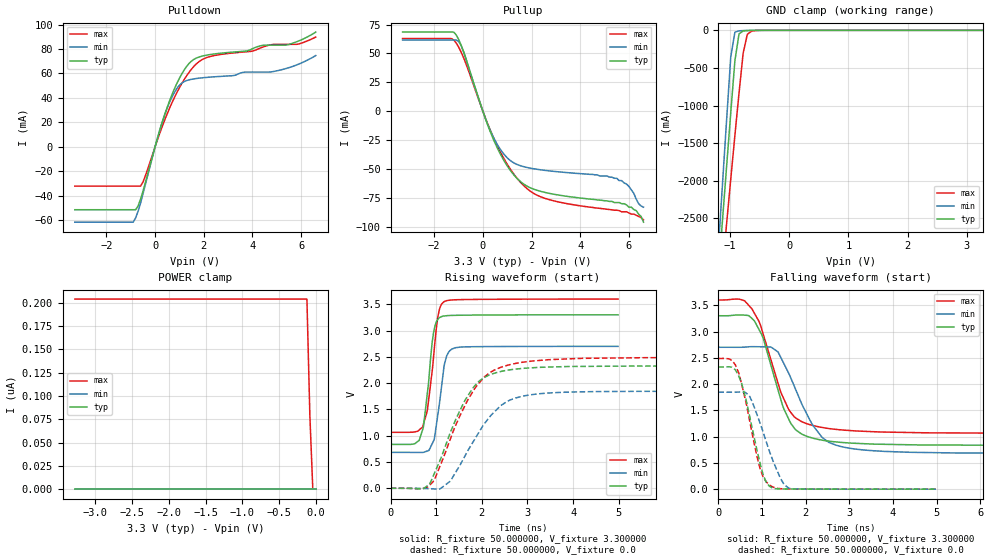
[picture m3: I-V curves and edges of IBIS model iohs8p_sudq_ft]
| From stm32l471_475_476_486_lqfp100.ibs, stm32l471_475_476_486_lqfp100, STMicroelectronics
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|   Model iohs8p_sudq_ft
[Model]  iohs8p_sudq_ft
Model_type I/O
Polarity   Non-Inverting
Enable   Active-Low
Vinl =   0.990000V
Vinh =   2.310000V
Vmeas =  1.650000V
Cref =   30.000000pF
Rref =   100.000000M
Vref =   0.0V
C_comp   2.036400pF   1.984000pF   2.082300pF
[Temperature Range]   25.000000   -40.000000   0.125000k
[Pullup Reference]   3.300000V   2.700000V   3.600000V
[Pulldown Reference]   0.0V   0.0V   0.0V
[POWER Clamp Reference]   3.300000V   2.700000V   3.600000V
[GND Clamp Reference]   0.0V   0.0V   0.0V
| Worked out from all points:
|   slope of the pulldown table from 0 to 0.495 V, typ, clamps not added: 15.4 ohm
|   slope of the pullup table from 0 to 0.495 V, typ, clamps not added: 18.1 ohm
|   GND clamp passes 1 mA (typ) near -0.60 V on its own axis
|   rising waveform, R_fixture 50.000000, V_fixture 3.300000: 20-80 % time 175ps typ, 184ps min, 191ps max; typ from 0.835 V to 3.3 V
|   rising waveform, R_fixture 50.000000, V_fixture 0.0: 20-80 % time 718ps typ, 830ps min, 808ps max; typ from 0 V to 2.33 V
|   falling waveform, R_fixture 50.000000, V_fixture 3.300000: 20-80 % time 564ps typ, 726ps min, 605ps max; typ from 3.3 V to 0.835 V
|   falling waveform, R_fixture 50.000000, V_fixture 0.0: 20-80 % time 381ps typ, 476ps min, 388ps max; typ from 2.33 V to 0 V
[Pulldown]
|Voltage   I(typ)   I(min)   I(max)
-3.3V     -51.63mA   -61.84mA   -32.32mA
-900mV    -51.63mA   -61.84mA   -32.32mA
-800mV    -51.63mA   -58.24mA   -32.32mA
-500mV    -36.51mA   -38.71mA   -28.96mA
400mV     26.66mA    26.58mA    22.18mA
800mV     47.72mA    44.74mA    40.6mA
1.1V      59.79mA    52.18mA    51.93mA
1.5V      70.22mA    55.24mA    63.66mA
2.1V      74.97mA    56.75mA    72.88mA
4.9V      83.19mA    61.75mA    83.83mA
5.9V      86.64mA    67.67mA    84.15mA
6.6V      93.9mA     74.68mA    89.84mA
[Pullup]
|Voltage   I(typ)   I(min)   I(max)
-3.3V     68.52mA    61.65mA    62.96mA
-1.1V     66.11mA    61.65mA    59.23mA
-800mV    51.99mA    51.74mA    46.62mA
100mV     -6.166mA   -5.972mA   -5.649mA
600mV     -32.08mA   -29.08mA   -30.29mA
1.2V      -53.2mA    -43.76mA   -52.32mA
1.9V      -65.77mA   -49.03mA   -68.4mA
3.1V      -72.48mA   -52.41mA   -78.44mA
5.5V      -79mA      -58mA      -85.6mA
6V        -83mA      -65mA      -88mA
6.3V      -86mA      -76mA      -90mA
6.6V      -96mA      -83mA      -94mA
[GND_clamp]
|Voltage   I(typ)   I(min)   I(max)
-3.3V     -9.812A    -9.822A    -9.937A
-1.2V     -3.251A    -2.905A    -3.763A
-1.13V    -2.527A    -2.046A    -3.165A
-1.06V    -1.808A    -1.191A    -2.57A
-990mV    -1.097A    -352.6mA   -1.979A
-920mV    -404.2mA   -25.08mA   -1.398A
-850mV    -46.53mA   -6.503mA   -832.3mA
-780mV    -8.496mA   -3.578mA   -302.4mA
-710mV    -3.383mA   -1.716mA   -53.8mA
-640mV    -1.589mA   -553.8uA   -11.72mA
-360mV    -2.023uA   0A         -84.67uA
3.28V     0A         0A         0A
[POWER_clamp]
|Voltage   I(typ)   I(min)   I(max)
-3.28V    0A         0A         204.1nA
-120mV    0A         0A         204.1nA
-80mV     0A         0A         79.47nA
-40mV     0A         0A         0A
0V        0A         0A         0A
[Ramp]
| variable   typ   min   max
dV/dt_r  1.39476/0.71674n   1.10718/0.82878n   1.49076/0.80690n
dV/dt_f  1.47901/0.56356n   1.21004/0.72569n   1.52124/0.60476n
R_load = 50.000000
[Rising Waveform]
R_fixture= 50.000000
V_fixture= 3.300000
V_fixture_min= 2.700000
V_fixture_max= 3.600000
|time   V(typ)   V(min)   V(max)
0s        835mV      683.3mV    1.065V
530.5ps   848.1mV    682.1mV    1.073V
700.7ps   1.11V      682.9mV    1.164V
810.8ps   1.844V     710.6mV    1.513V
940.9ps   2.954V     899mV      2.484V
1.041ns   3.221V     1.431V     3.281V
1.171ns   3.277V     2.318V     3.549V
1.281ns   3.286V     2.6V       3.577V
1.532ns   3.292V     2.686V     3.589V
4.985ns   3.3V       2.7V       3.6V
[Rising Waveform]
R_fixture= 50.000000
V_fixture= 0.0
V_fixture_min= 0.0
V_fixture_max= 0.0
|time   V(typ)   V(min)   V(max)
0s        24.38uV    -1.232uV   39.9uV
734.1ps   1.035mV    -3.343mV   -313.8uV
934.3ps   232.5mV    -11.62mV   128.5mV
1.101ns   566.2mV    -1.634mV   458.9mV
1.301ns   1.044V     130.8mV    917.4mV
1.602ns   1.625V     568.3mV    1.524V
1.902ns   2.007V     1.016V     1.962V
2.402ns   2.22V      1.563V     2.296V
2.803ns   2.273V     1.731V     2.385V
16.62ns   2.325V     1.845V     2.485V
[Falling Waveform]
R_fixture= 50.000000
V_fixture= 3.300000
V_fixture_min= 2.700000
V_fixture_max= 3.600000
|time   V(typ)   V(min)   V(max)
0s        3.3V       2.7V       3.6V
600.6ps   3.311V     2.703V     3.586V
834.2ps   3.192V     2.711V     3.336V
1.034ns   2.857V     2.709V     2.933V
1.368ns   1.888V     2.611V     2.016V
1.768ns   1.132V     1.904V     1.356V
2.336ns   938.9mV    1.031V     1.181V
2.936ns   882.5mV    789.5mV    1.12V
4.371ns   845.1mV    702.1mV    1.078V
16.62ns   835mV      683.3mV    1.065V
[Falling Waveform]
R_fixture= 50.000000
V_fixture= 0.0
V_fixture_min= 0.0
V_fixture_max= 0.0
|time   V(typ)   V(min)   V(max)
0s        2.325V     1.845V     2.485V
310.3ps   2.32V      1.845V     2.45V
450.5ps   2.187V     1.847V     2.245V
710.7ps   1.414V     1.775V     1.331V
951ps     511.3mV    1.267V     407.6mV
1.031ns   264.5mV    1.075V     230.5mV
1.181ns   51.28mV    698.8mV    72.53mV
1.431ns   5.2mV      195.2mV    8.721mV
1.622ns   3.374mV    16.99mV    4.414mV
4.985ns   24.38uV    -1.232uV   39.9uV
